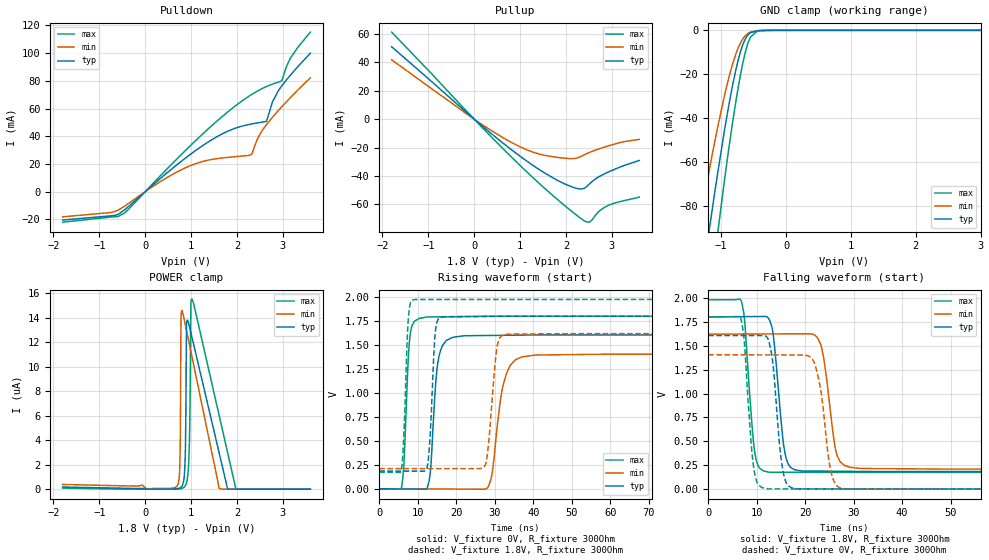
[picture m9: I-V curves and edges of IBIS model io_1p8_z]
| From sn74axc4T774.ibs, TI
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|   io_1p8_z Model
[Model]   io_1p8_z
Model_type   I/O
Polarity   Non-Inverting
Enable   Active-Low
Vinl = 0.63
Vinh = 1.17
Vmeas = 0.9
Vref = 0
Cref = 2pF
Rref = 100000
|   typ   min   max
C_comp   2.803pF   2.059pF   3.293pF
[Model spec]
|subparameter
Vinl   0.63   0.567   0.693
Vinh   1.17   1.053   1.287
| Where Nom  PVT is Nominal Process, 1.8V, 27C
|   Fast PVT is Strong Process,  1.98V, -40C
|   Slow PVT is Weak Process,   1.62V, 130C
[Voltage Range]   1.8   1.62   1.98
|Junction Temperature
[Temperature Range]   27   130   -40
[Pullup Reference]   1.8   1.62   1.98
[Pulldown Reference]   -0   0   -0
[Power Clamp Reference]   1.8   1.62   1.98
[GND Clamp Reference]   0   0   0
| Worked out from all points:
|   slope of the pulldown table from 0 to 0.27 V, typ, clamps not added: 34.5 ohm
|   slope of the pullup table from 0 to 0.27 V, typ, clamps not added: 36.5 ohm
|   GND clamp passes 1 mA (typ) near -0.54 V on its own axis
|   falling waveform, V_fixture 1.8V, R_fixture 300Ohm: 20-80 % time 1.74ns typ, 2.08ns min, 1.54ns max; typ from 1.8 V to 0.184 V
|   rising waveform, V_fixture 0V, R_fixture 300Ohm: 20-80 % time 1.57ns typ, 2.78ns min, 1.14ns max; typ from 0 V to 1.61 V
|   rising waveform, V_fixture 1.8V, R_fixture 300Ohm: 20-80 % time 1.13ns typ, 1.72ns min, 973ps max; typ from 0.184 V to 1.8 V
|   falling waveform, V_fixture 0V, R_fixture 300Ohm: 20-80 % time 1.62ns typ, 2.08ns min, 1.48ns max; typ from 1.61 V to 0 V
[Pulldown]
|   Voltage   I(typ)   I(min)   I(max)
-1.8V     -20.45mA   -18.15mA   -22.02mA
-671.4mV  -17.14mA   -14.4mA    -18.13mA
-444.6mV  -13.01mA   -10.37mA   -15.3mA
986.4mV   26.99mA    18.81mA    33.29mA
1.732V    42.62mA    24.55mA    55.72mA
2.326V    48.94mA    27.14mA    70.28mA
2.434V    49.59mA    37.14mA    72.41mA
2.639V    50.71mA    48.22mA    75.86mA
2.774V    64.75mA    53.7mA     77.7mA
2.974V    76.22mA    61.16mA    79.94mA
3.168V    84.27mA    68mA       96.51mA
3.6V      100mA      82.21mA    115.2mA
[GND Clamp]
|   Voltage   I(typ)   I(min)   I(max)
-1.8V     -227.7mA   -173.3mA   -280.5mA
-1.314V   -118.5mA   -85.12mA   -156mA
-1.211V   -96.81mA   -68.22mA   -130.5mA
-1.114V   -76.99mA   -53.06mA   -106.8mA
-1.06V    -66.38mA   -45.06mA   -94mA
-898.2mV  -36.91mA   -23.54mA   -57.37mA
-774mV    -18.07mA   -10.82mA   -32.58mA
-671.4mV  -6.964mA   -4.128mA   -15.65mA
-574.2mV  -1.723mA   -1.197mA   -4.839mA
-444.6mV  -206.1uA   -178.2uA   -421.8uA
-342mV    -62.95uA   -50.11uA   -87.95uA
3.6V      0A         0A         0A
[Pullup]
|   Voltage   I(typ)   I(min)   I(max)
-1.8V     50.91mA    41.74mA    61.18mA
84.6mV    -2.344mA   -1.871mA   -2.849mA
538.2mV   -14.51mA   -11.29mA   -17.83mA
959.4mV   -25.07mA   -18.79mA   -31.25mA
1.37V     -34.39mA   -24.1mA    -43.74mA
1.748V    -41.81mA   -26.58mA   -54.61mA
2.169V    -48.03mA   -27.74mA   -65.9mA
2.39V     -48.72mA   -25.27mA   -71.29mA
2.525V    -45.19mA   -23.25mA   -72.19mA
2.725V    -40.4mA    -20.86mA   -64.65mA
2.979V    -36.4mA    -18.28mA   -59.89mA
3.6V      -29.04mA   -14.25mA   -54.84mA
[POWER Clamp]
|   Voltage   I(typ)   I(min)   I(max)
-1.8V     171.8nA    383.4nA    88.28nA
689.4mV   39.1nA     223nA      575.5pA
754.2mV   97.12nA    1.895uA    18.8nA
781.2mV   159nA      14.01uA    37.55nA
867.6mV   2.112uA    13.55uA    243nA
900mV     13.42uA    12.97uA    522.5nA
959.4mV   13.35uA    11.9uA     3.252uA
997.2mV   12.76uA    11.22uA    15.28uA
1.013V    12.5uA     10.93uA    15.53uA
1.613V    2.958uA    63.04nA    6.012uA
1.975V    0A         0A         50.55nA
3.6V      0A         0A         0A
[Ramp]
R_load = 300
|   typ   min   max
dV/dt_r   0.96337/1.5612e-09   0.843144/2.72911e-09   1.08069/1.12652e-09
dV/dt_f   0.969407/1.72299e-09   0.846054/2.07462e-09   1.08473/1.52931e-09
[Falling Waveform]
V_fixture = 1.8V
V_fixture_min = 1.62V
V_fixture_max = 1.98V
R_fixture = 300Ohm
C_fixture = 0F
|   Time   V(typ)   V(min)   V(max)
0s        1.8V       1.62V      1.98V
6.828ns   1.803V     1.621V     1.966V
9.654ns   1.805V     1.622V     370.7mV
12.62ns   1.768V     1.623V     176.3mV
15.89ns   361.8mV    1.623V     176.3mV
19.23ns   190.6mV    1.624V     176.3mV
23.24ns   188.5mV    1.506V     176.2mV
26.7ns    187.3mV    337.5mV    176.2mV
31.43ns   185.5mV    216.6mV    176.2mV
500ns     184.3mV    209.9mV    172.1mV
[Rising Waveform]
V_fixture = 0V
V_fixture_min = 0V
V_fixture_max = 0V
R_fixture = 300Ohm
C_fixture = 0F
|   Time   V(typ)   V(min)   V(max)
0s        160.4nV    874.6nV    70.32nV
5.765ns   -1.991mV   -880.6uV   11.26mV
8.089ns   -2.794mV   -1.236mV   1.625V
12.38ns   4.247mV    -1.892mV   1.792V
15.57ns   1.391V     -2.379mV   1.794V
21.67ns   1.596V     -3.312mV   1.797V
28.31ns   1.6V       22.26mV    1.801V
32.93ns   1.602V     1.189V     1.801V
40.21ns   1.605V     1.394V     1.801V
500ns     1.606V     1.405V     1.801V
[Rising Waveform]
V_fixture = 1.8V
V_fixture_min = 1.62V
V_fixture_max = 1.98V
R_fixture = 300Ohm
C_fixture = 0F
|   Time   V(typ)   V(min)   V(max)
0s        184.3mV    209.9mV    172.1mV
5.743ns   184.4mV    210.1mV    194.5mV
7.562ns   184.4mV    210.1mV    1.78V
9.208ns   184.4mV    210.2mV    1.975V
12.55ns   247.8mV    210.3mV    1.975V
14.6ns    1.648V     210.3mV    1.975V
16.74ns   1.795V     210.4mV    1.975V
27.57ns   1.798V     252.5mV    1.976V
33.46ns   1.799V     1.615V     1.976V
500ns     1.8V       1.62V      1.98V
[Falling Waveform]
|Gnd
V_fixture = 0V
V_fixture_min = 0V
V_fixture_max = 0V
R_fixture = 300Ohm
C_fixture = 0F
|   Time   V(typ)   V(min)   V(max)
0s        1.606V     1.405V     1.801V
6.73ns    1.605V     1.404V     1.786V
9.483ns   1.605V     1.404V     191.8mV
12.38ns   1.563V     1.403V     2.39mV
15.48ns   176.4mV    1.403V     2.375mV
18.45ns   2.228mV    1.403V     2.36mV
21.8ns    2.212mV    1.331V     2.344mV
25.47ns   2.195mV    152.2mV    2.326mV
28.31ns   2.182mV    3.049mV    2.312mV
500ns     179.5nV    909.3nV    81nV
